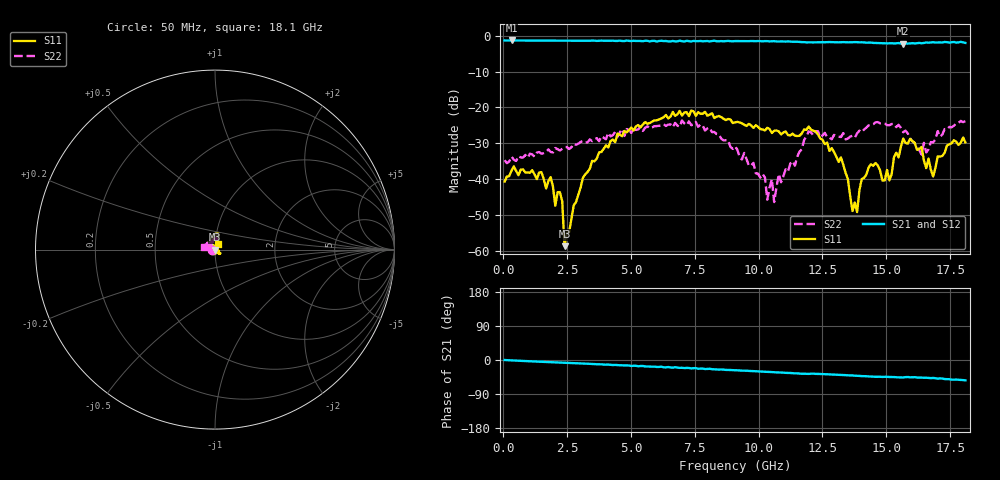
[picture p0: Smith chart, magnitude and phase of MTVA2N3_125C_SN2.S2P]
! Network Analyzer HP8720D.06.14 Serial No. US36140669
! 11 May 2005  13:02:58
! Frequency  S11  S21  S12  S22
# HZ  S  DB R 50
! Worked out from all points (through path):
!   201 points, 50 MHz to 18.1 GHz, reference 50 ohm
!   highest |S21| = -1.31 dB at 320.8 MHz (marker M1); lowest = -2.2 dB at 15.66 GHz (marker M2)
!   group delay of S21, straight-line fit = 8.1 ps
!   lowest |S11| = -58.7 dB at 2.397 GHz (marker M3), VSWR 1.00, Z = 50.1 - j0.0572 ohm
!   |S11| at or under -10 dB: start of sweep to end of sweep
!   |S22| runs from -46.4 to -23.6 dB; largest |S21 - S12| = 0.029
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5e7  -40.69 -162.3  -1.32 -0.0  -1.33 -0.7  -34.76 -172.0
3.2075e8  -37.62 -168.0  -1.31 -1.0  -1.32 -1.5  -33.73 -170.7
1.855e9  -39.46 -129.0  -1.36 -5.7  -1.35 -6.1  -32.45 172.3
2.0355e9  -47.43 -123.5  -1.36 -6.2  -1.36 -6.6  -31.33 173.0
2.30625e9  -46.20 -92.9  -1.37 -7.1  -1.36 -7.4  -31.57 166.5
2.3965e9  -58.74 -29.6  -1.36 -7.2  -1.35 -7.8  -31.10 162.3
3.1185e9  -39.63 61.8  -1.37 -9.3  -1.37 -10.0  -29.35 155.4
6.09675e9  -23.35 80.1  -1.47 -18.3  -1.40 -18.6  -25.14 93.1
9.075e9  -24.21 105.6  -1.49 -27.0  -1.46 -27.6  -30.90 70.5
1.024825e10  -26.42 120.2  -1.49 -31.1  -1.50 -31.4  -39.58 50.4
1.03385e10  -25.70 121.3  -1.51 -31.2  -1.51 -31.9  -45.78 55.5
1.0519e10  -27.15 126.0  -1.54 -32.0  -1.54 -32.5  -40.04 80.8
1.060925e10  -26.53 123.1  -1.50 -32.5  -1.53 -33.1  -46.43 73.4
1.078975e10  -26.70 131.0  -1.61 -32.9  -1.55 -33.3  -38.58 118.7
1.21435e10  -26.54 121.8  -1.85 -36.0  -1.81 -36.7  -27.84 125.5
1.32265e10  -33.97 113.9  -1.82 -39.5  -1.81 -40.0  -28.27 133.5
1.367775e10  -48.92 -149.9  -1.81 -40.7  -1.77 -41.2  -27.91 151.1
1.439975e10  -35.86 -113.1  -1.91 -43.6  -1.89 -44.0  -24.92 163.6
1.512175e10  -40.38 -71.5  -2.11 -44.9  -2.04 -45.0  -24.99 150.2
1.566325e10  -28.71 -33.7  -2.22 -46.2  -2.18 -45.9  -26.93 140.4
1.68365e10  -39.28 27.7  -1.79 -47.3  -1.75 -48.9  -29.79 -179.9
1.81e10  -29.75 61.4  -2.00 -53.6  -1.93 -55.2  -23.85 169.5
